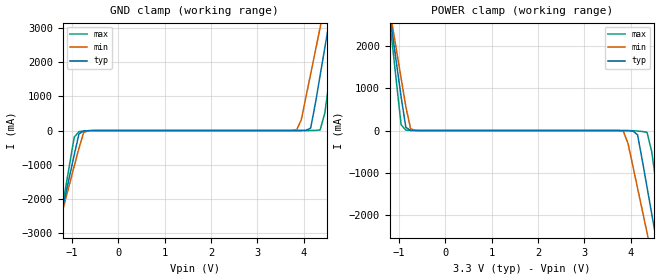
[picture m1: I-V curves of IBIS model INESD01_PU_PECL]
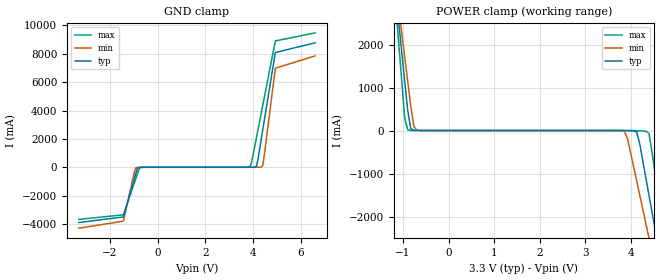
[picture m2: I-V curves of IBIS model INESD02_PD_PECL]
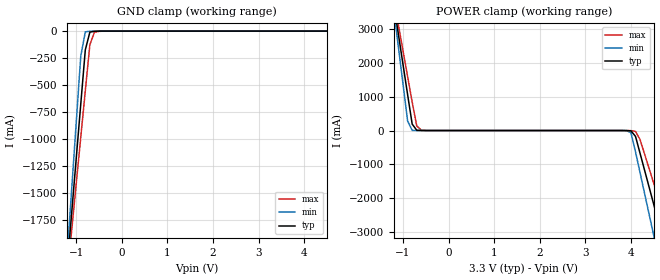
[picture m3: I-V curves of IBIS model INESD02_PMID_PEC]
|   This file is an IBIS representation of the   |
|   Integrated Device Technology, Inc.   |
|   ICS873996   |
|   DIFFERENTIAL-TO-3.3V LVPECL ZERO DELAY/MULTIPLIER/DIVIDER   |
[IBIS Ver]   4.1
[File name]   873996_3v3.ibs
[File Rev]   1.0
[Date]   13 Jan 2009 | Last modified
[Source]   Originated at Integrated Devices Technology, Inc.
[Disclaimer]
IDT hereby grants the user of this IBIS model a non-exclusive,
nontransferable license to use this IBIS model under the following terms.
Before using this IBIS model, the user should read this license.
If the user does not accept these terms,  the IBIS model should be
returned to IDT within 30 days.
   The user is granted this license only to use the IBIS model and
is not granted rights to sell, load, rent, lease or license the IBIS
model in whole or in part, or in modified form to anyone other than
user. User may modify the IBIS model to suit its specific
applications but rights to derivative works and such modifications
shall belong to IDT.
   This IBIS model is provided on an "AS IS" basis and IDT makes
absolutely no warranty with respect to the information contained
herein. IDT DISCLAIMS AND CUSTOMER WAIVES ALL WARRANTIES, EXPRESS
OR IMPLIED, INCLUDING WARRANTIES OF MERCHANTABILITY OR FITNESS FOR
A PARTICULAR PURPOSE. The entire risk as to quality and performance
is with the Customer. ACCORDINGLY, IN NO EVENT SHALL THE COMPANY BE
LIABLE FOR ANY DAMAGES, WHETHER IN CONTRACT OR TORT,INCLUDING ANY
LOST PROFITS OR OTHER INCIDENTAL, CONSEQUENTIAL, EXEMPLARY, OR
PUNITIVE DAMAGES ARISING OUT OF THE USE OR APPLICATION OF THE IBIS
model provided in this package. Further, IDT reserves the right to
make changes without notice to any product herein to improve
reliability, function, or design. IDT does not convey any license
under patent rights or any other intellectual property rights,
including those of third parties.
   IDT is not obligated to provide maintenance or support
for the licensed IBIS model.
[Copyright]   Copyright 2005 by Integrated Device Technology, Inc.
[Component]   ICS873996Y
[Manufacturer] Integrated Devices Technology, Inc.
[Package]
|TQFP48 Epad
|lead + wire   typ   min   max
R_pkg   86.05m   81.2m   90.9m
L_pkg   2.653n   2.410n   2.895n
C_pkg   0.407p   0.381p   0.433p
[Pin] signal_name   model_name   R_pin   L_pin   C_pin
1   PLL_SEL   INESD01_PU_PECL   90.90m   2.895n   0.433p
2   nMR   INESD01_PU_PECL   88.96m   2.798n   0.428p
3   nINIT   INESD01_PU_PECL   87.02m   2.701n   0.423p
4   VEE   GND   85.08m   2.604n   0.417p
5   CLK0   INESD02_PD_PECL   83.40m   2.507n   0.412p
6   nCLK0   INESD02_PD_PECL   81.20m   2.410n   0.407p
7   CLK1   INESD02_PD_PECL   81.20m   2.410n   0.407p
8   nCLK1   INESD02_PMID_PEC   83.40m   2.507n   0.412p
9   EXT_FB   INESD02_PD_PECL   85.08m   2.604n   0.417p
10   nEXT_FB   INESD02_PMID_PEC   87.02m   2.701n   0.423p
11   SEL_CLK   INESD01_PD_PECL   88.96m   2.798n   0.428p
12   BW   INESD02_3LEVEL   90.90m   2.895n   0.433p
13   VCC   POWER   90.90m   2.895n   0.433p
14   NB0   INESD01_PU_PECL   88.96m   2.798n   0.428p
15   NB1   INESD01_PU_PECL   87.02m   2.701n   0.423p
16   NB2   INESD01_PU_PECL   85.08m   2.604n   0.417p
17   VEE   GND   83.40m   2.507n   0.412p
18   NA0   INESD01_PU_PECL   81.20m   2.410n   0.407p
19   NA1   INESD01_PU_PECL   81.20m   2.410n   0.407p
20   NA2   INESD01_PU_PECL   83.40m   2.507n   0.412p
21   VCCO_B   POWER   85.08m   2.604n   0.417p
22   nQB2   ONF01_PECL01_ABI   87.02m   2.701n   0.423p
23   QB2   ONF01_PECL01_ABI   88.96m   2.798n   0.428p
24   nQB1   ONF01_PECL01_ABI   90.90m   2.895n   0.433p
25   QB1   ONF01_PECL01_ABI   90.90m   2.895n   0.433p
26   nQB0   ONF01_PECL01_ABI   88.96m   2.798n   0.428p
27   QB0   ONF01_PECL01_ABI   87.02m   2.701n   0.423p
28   VCCO_B   POWER   85.08m   2.604n   0.417p
29   VCCO_A   POWER   83.40m   2.507n   0.412p
30   nQA2   ONF01_PECL01_ABI   81.20m   2.410n   0.407p
31   QA2   ONF01_PECL01_ABI   81.20m   2.410n   0.407p
32   nAQ1   ONF01_PECL01_ABI   83.40m   2.507n   0.412p
33   QA1   ONF01_PECL01_ABI   85.08m   2.604n   0.417p
34   nQA0   ONF01_PECL01_ABI   87.02m   2.701n   0.423p
35   QA0   ONF01_PECL01_ABI   88.96m   2.798n   0.428p
36   VCCO_A   POWER   90.90m   2.895n   0.433p
37   VCCO_FB   POWER   90.90m   2.895n   0.433p
38   QFB   ONF01_PECL01_ABI   88.96m   2.798n   0.428p
39   nQFB   ONF01_PECL01_ABI   87.02m   2.701n   0.423p
40   VCCA   POWER   85.08m   2.604n   0.417p
41   NFB0   INESD01_PU_PECL   83.40m   2.507n   0.412p
42   NFB1   INESD01_PU_PECL   81.20m   2.410n   0.407p
43   NFB2   INESD01_PU_PECL   81.20m   2.410n   0.407p
44   CLK_INDICATOR   COUT10_15_OHM   83.40m   2.507n   0.412p
45   INP0BAD   COUT10_15_OHM   85.08m   2.604n   0.417p
46   INP1BAD   COUT10_15_OHM   87.02m   2.701n   0.423p
47   VCC   POWER   88.96m   2.798n   0.428p
48   MAN_OVERRIDE   INESD01_PD_PECL   90.90m   2.895n   0.433p
[Diff Pin]  inv_pin  vdiff tdelay_typ tdelay_min  tdelay_max
|Output
23   22   NA   0   0   0
25   24   NA   0   0   0
27   26   NA   0   0   0
31   30   NA   0   0   0
33   32   NA   0   0   0
35   34   NA   0   0   0
38   39   NA   0   0   0
|Input
5   6   0.15   0   0   0
7   8   0.15   0   0   0
9   10   0.15   0   0   0
| Models and submodels in the file (7): INESD01_PU_PECL (Input), INESD02_PD_PECL (Input), INESD02_PMID_PEC (Input), INESD01_PD_PECL (Input), INESD02_3LEVEL (Input), ONF01_PECL01_ABI (Output_ECL), COUT10_15_OHM (Output)
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[Model]   INESD01_PU_PECL
Model_type  Input
Polarity   Non-Inverting
Vinl = 0.8V
Vinh = 2.0V
|   typ   min   max
C_comp   2pF   1.5pF   2.5pF
|   typ   min   max
[Voltage range]  3.3V   3.15V   3.45V
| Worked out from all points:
|   GND clamp passes 1 mA (typ) near -0.55 V on its own axis
|   POWER clamp passes 1 mA (typ) near -0.67 V on its own axis
[GND_clamp]
|Voltage   I(typ)   I(min)   I(max)
-3.3V     -15.3A     -13.19A    -18.82A
-1.361V   -3.24A     -3.145A    -3.432A
-1.259V   -2.606A    -2.617A    -2.622A
-952.6mV  -705.4mA   -1.038A    -192.5mA
-850.5mV  -99.96mA   -513.6mA   -31.29mA
-646.4mV  -3.852mA   -3.611mA   -8.361mA
3.844V    64.83uA    13.07mA    7.183uA
4.151V    73.26mA    1.652A     800.8uA
4.355V    1.607A     3.003A     15.37mA
4.559V    3.233A     4.356A     1.553A
4.763V    4.861A     5.711A     3.635A
6.6V      19.56A     17.94A     22.42A
[POWER_clamp]
|Voltage   I(typ)   I(min)   I(max)
-3.3V     19.56A     16.84A     24.11A
-1.259V   3.233A     3.262A     3.235A
-1.157V   2.419A     2.586A     2.194A
-952.6mV  795.8mA    1.236A     137.7mA
-850.5mV  73.26mA    563.1mA    8.081mA
-646.4mV  471.5uA    1.942mA    367.2uA
3.844V    -890.5uA   -18.21mA   -111uA
4.151V    -99.96mA   -1.362A    -11.88mA
4.355V    -1.338A    -2.415A    -41.77mA
4.559V    -2.606A    -3.47A     -1.313A
4.763V    -3.875A    -4.526A    -2.933A
6.6V      -15.3A     -14.05A    -17.51A
[Model]   INESD02_PD_PECL
Model_type  Input
Polarity   Non-Inverting
Vinl = 0.8V
Vinh = 2.0V
|   typ   min   max
C_comp   2pF   1.5pF   2.5pF
|   typ   min   max
[Voltage range]  3.3V   3.15V   3.45V
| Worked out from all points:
|   GND clamp passes 1 mA (typ) near -0.59 V on its own axis
|   POWER clamp passes 1 mA (typ) near -0.70 V on its own axis
[GND_clamp]
-3.3V     -3.894A    -4.294A    -3.674A
-1.434V   -3.506A    -3.799A    -3.352A
-974.8mV  -794.1mA   -331.5mA   -1.096A
-909.1mV  -407.1mA   -35.25mA   -774.3mA
-777.8mV  -10.55mA   -10.84mA   -133.1mA
-646.5mV  -1.912mA   -4.151mA   -2.665mA
3.884V    141.8uA    72.03uA    57.99mA
3.95V     342.2uA    75.94uA    423.8mA
4.146V    78.32mA    440.9uA    2.118A
4.409V    2.651A     112.4mA    4.38A
4.934V    8.093A     6.984A     8.908A
6.6V      8.773A     7.854A     9.475A
[POWER_clamp]
-3.3V     6.7A       6.327A     7.39A
-1.165V   3.23A      3.44A      2.951A
-1.031V   1.843A     2.286A     1.176A
-963.9mV  1.149A     1.709A     289.6mA
-896.9mV  456.5mA    1.133A     15.4mA
-695.9mV  792.2uA    10.73mA    555.6uA
3.861V    -556.7uA   -26.14mA   -39.45uA
4.129V    -41.85mA   -1.19A     -4.904mA
4.33V     -1.119A    -2.176A    -17.86mA
4.531V    -2.305A    -3.163A    -1.019A
4.732V    -3.492A    -4.151A    -2.536A
6.6V      -5.075A    -5.468A    -4.558A
[Model]   INESD02_PMID_PEC
Model_type   Input
Polarity   Non-Inverting
Vinl = 0.8V
Vinh = 2.0V
|   typ   min   max
C_comp   2pF   1.5pF   2.5pF
|   typ   min   max
[Voltage range]  3.3V   3.15V   3.45V
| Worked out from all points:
|   GND clamp passes 1 mA (typ) near -0.54 V on its own axis
|   POWER clamp passes 1 mA (typ) near -0.60 V on its own axis
[GND_clamp]
|Voltage   I(typ)   I(min)   I(max)
-3.3V     -12.83A    -15.14A    -11.37A
-1.2V     -2.195A    -2.092A    -2.281A
-1.1V     -1.689A    -1.472A    -1.849A
-900mV    -678.6mA   -232.7mA   -984.9mA
-800mV    -174mA     -7.255mA   -553.3mA
-700mV    -9.789mA   -1.13mA    -126.1mA
-600mV    -1.72mA    -254.4uA   -11.17mA
-500mV    -427uA     -99.72uA   -2.216mA
6.6V      76.52uA    70.16uA    79.2uA
[POWER_clamp]
|Voltage   I(typ)   I(min)   I(max)
-3.3V     22.38A     26.45A     19.82A
-1.2V     3.723A     3.545A     3.874A
-1.1V     2.836A     2.457A     3.116A
-900mV    1.063A     281mA      1.601A
-800mV    191.6mA    5.071mA    844mA
-600mV    678.1uA    76.63uA    10.7mA
3.9V      -1.629mA   -3.157mA   -831.1uA
4.1V      -173.9mA   -635.2mA   -23.94mA
4.5V      -2.195A    -3.116A    -1.568A
4.7V      -3.206A    -4.358A    -2.433A
4.9V      -4.218A    -5.6A      -3.298A
6.6V      -12.83A    -16.16A    -10.66A
